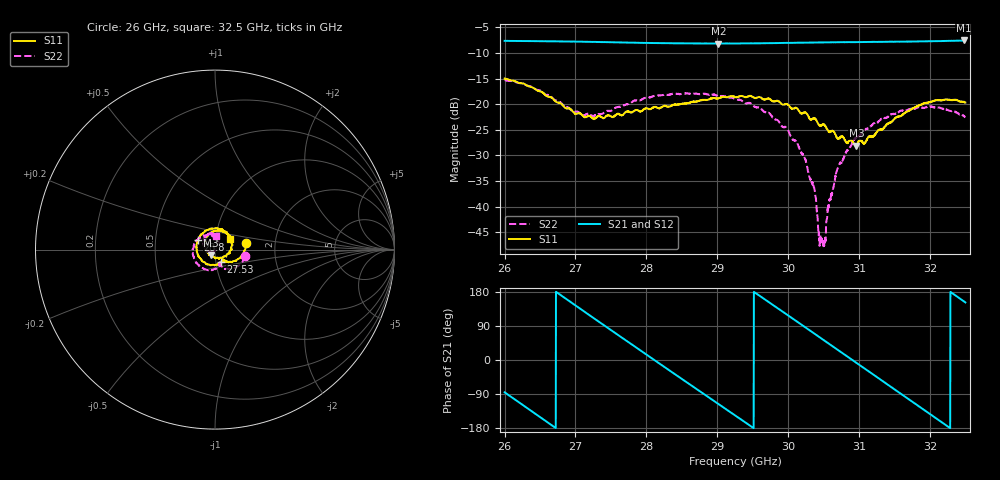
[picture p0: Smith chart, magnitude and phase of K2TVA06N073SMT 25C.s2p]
!Keysight Technologies,N5247B,US57180393,A.17.35.14
!Date: Wednesday, May 07, 2025 10:43:43
!Correction: S11(C  2-Port  )
!S21(C  2-Port  )
!S12(C  2-Port  )
!S22(C  2-Port  )
!S2P File: Measurements: S11, S21, S12, S22:
# Hz S  RI  R 50
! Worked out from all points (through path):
!   2001 points, 26 GHz to 32.5 GHz, reference 50 ohm
!   highest |S21| = -7.55 dB at 32.47 GHz (marker M1); lowest = -8.2 dB at 29.02 GHz (marker M2)
!   lowest |S11| = -28.1 dB at 30.96 GHz (marker M3), VSWR 1.08, Z = 47.5 - j2.94 ohm
!   |S11| at or under -10 dB: start of sweep to end of sweep
!   |S22| runs from -47.7 to -15.3 dB; largest |S21 - S12| = 0.0027
!   S11 on the Smith chart (normalised r, x): 26 GHz: 1.42, +0.11; 27.53 GHz: 1.06, -0.14; 28.8 GHz: 0.82, +0.09; 32.5 GHz: 1.17, +0.15
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2.6e10  0.1737 0.0379  0.0341 -0.4143  0.0343 -0.4132  0.1685 -0.0348
2.658825e10  0.1023 -0.064  -0.392 -0.1258  -0.391 -0.1261  0.061 -0.1069
2.70855e10  0.0515 -0.0603  -0.2775 0.2994  -0.2763 0.2984  0.0269 -0.0744
2.7534e10  0.033 -0.068  0.1077 0.3876  0.1071 0.3863  0.0262 -0.0856
2.816775e10  -0.0531 -0.0747  0.3923 -0.0503  0.3904 -0.0497  -0.0446 -0.1135
2.880475e10  -0.0951 0.0556  0.00613 -0.3918  0.00666 -0.391  -0.1228 -0.0286
2.9016e10  -0.0626 0.0949  -0.1716 -0.3508  -0.1717 -0.3508  -0.1192 0.0124
2.925e10  -0.0133 0.1165  -0.3253 -0.2188  -0.3246 -0.2184  -0.0989 0.053
2.960425e10  0.0649 0.0971  -0.3856 0.0785  -0.3844 0.0782  -0.0415 0.0825
2.998125e10  0.0974 0.0247  -0.1981 0.3442  -0.198 0.3429  0.0119 0.0567
3.022175e10  0.0799 -0.0194  0.00795 0.399  0.00812 0.3977  0.0193 0.0243
3.03355e10  0.0638 -0.0329  0.1092 0.3849  0.1094 0.3834  0.0147 0.009
3.044925e10  0.0469 -0.0408  0.2038 0.3444  0.2045 0.3435  0.00401 -0.00132
3.0498e10  0.0421 -0.0472  0.2417 0.3207  0.2402 0.319  0.0019 -0.00364
3.057925e10  0.0274 -0.0461  0.2966 0.271  0.2953 0.2703  -0.00758 -0.0088
3.06995e10  0.0104 -0.0448  0.3594 0.1819  0.3582 0.1813  -0.0214 -0.00995
3.096275e10  -0.0247 -0.0309  0.4006 -0.0524  0.3997 -0.052  -0.0473 -0.00254
3.141775e10  -0.0581 0.0289  0.1613 -0.3741  0.161 -0.3726  -0.0637 0.0418
3.185975e10  -0.0193 0.0963  -0.2313 -0.3394  -0.23 -0.3387  -0.047 0.081
3.2175e10  0.0402 0.102  -0.4004 -0.1047  -0.4001 -0.1048  -0.017 0.0889
3.2474e10  0.0825 0.0655  -0.3812 0.1745  -0.3791 0.173  0.00607 0.0767
3.25e10  0.0833 0.0616  -0.3699 0.1971  -0.3694 0.1967  0.00617 0.074
